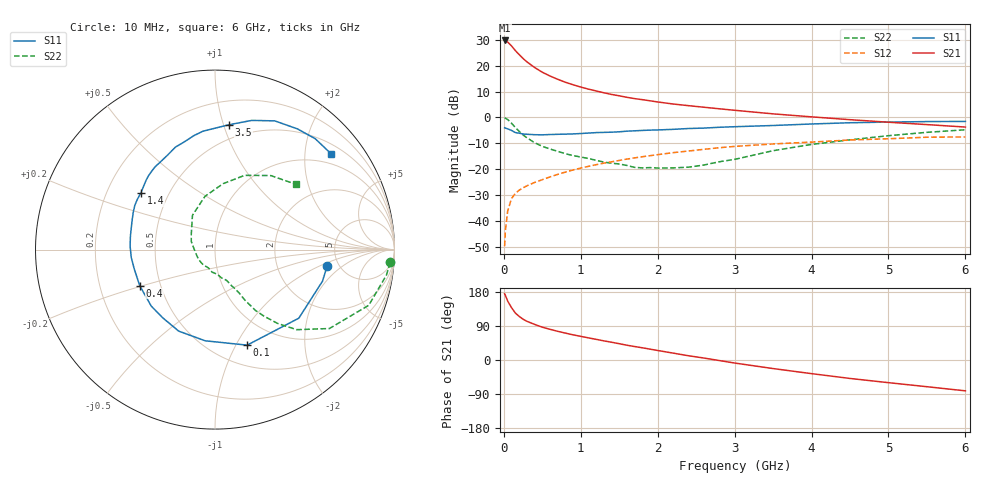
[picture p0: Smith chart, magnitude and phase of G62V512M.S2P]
! SIEMENS Small Signal Semiconductors
! BFG193
! Si NPN RF Bipolar Junction Transistor in SOT223
! VCE = 2.5 V  IC = 12 mA
! Common Emitter S-Parameters:  August  1996
# GHz  S  MA  R  50
!  f  S11  S21  S12  S22
! GHz  MAG  ANG  MAG  ANG  MAG  ANG  MAG  ANG
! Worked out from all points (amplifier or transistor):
!   36 points, 10 MHz to 6 GHz, reference 50 ohm
!   highest |S21| = 29.7 dB at 10 MHz (marker M1)
!   |S21| within 3 dB of that: start of sweep to 124.6 MHz
!   unconditionally stable (mu >= 1): 802.7 MHz to 2.628 GHz
!   at 250 MHz: K = 0.60, MSG = 24.9 dB, |S12| = -27.1 dB
!   at 1.4 GHz: K = 1.07, MAG = 11.4 dB, |S12| = -17.1 dB
!   at 6 GHz: K = 0.90, MSG = 1.9 dB, |S12| = -7.5 dB
!   S11 on the Smith chart (normalised r, x): 10 MHz: 4.05, -1.22; 100 MHz: 0.72, -1.11; 400 MHz: 0.38, -0.20; 1.4 GHz: 0.35, +0.30; 3.5 GHz: 0.38, +1.04; 6 GHz: 0.72, +2.61
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0.01  0.632 -8.2  30.51 174.7  0.0033 88.0  0.9787 -4.2
0.02  0.6242 -16.4  30.2 170.5  0.0066 84.7  0.966 -8.4
0.05  0.6034 -39.3  28.38 155.4  0.0157 73.2  0.9112 -19.9
0.1  0.5616 -71.4  23.92 138.1  0.0274 62.9  0.7744 -34.6
0.15  0.5111 -96.1  19.44 123.8  0.0344 55.8  0.6376 -44.4
0.2  0.4972 -114.0  16.25 115.0  0.0397 53.2  0.5396 -49.7
0.25  0.4787 -127.6  13.7 107.6  0.044 51.5  0.4595 -53.7
0.3  0.4746 -138.5  11.8 102.1  0.0481 51.7  0.4063 -56.4
0.4  0.4651 -154.4  9.191 93.9  0.0558 52.2  0.3259 -59.4
0.5  0.4625 -166.3  7.444 86.6  0.0631 52.0  0.2771 -60.9
0.6  0.4686 -174.6  6.301 81.0  0.0715 52.6  0.2464 -62.7
0.7  0.4733 177.7  5.442 75.7  0.0799 52.8  0.2223 -65.3
0.9  0.4815 165.8  4.267 66.4  0.0973 51.8  0.1839 -69.2
1.1  0.5003 155.6  3.516 58.4  0.1142 50.3  0.1616 -77.1
1.4  0.5199 142.5  2.776 46.9  0.1396 46.1  0.1314 -90.6
1.7  0.5528 132.3  2.308 35.5  0.1661 41.6  0.1091 -108.5
2.2  0.5899 116.4  1.818 18.2  0.2095 31.9  0.1066 -150.5
2.8  0.6463 100.4  1.469 -1.4  0.2607 19.4  0.1398 160.9
3.5  0.6996 83.7  1.173 -22.6  0.3083 2.9  0.2287 123.3
4.5  0.7907 65.1  0.906 -48.7  0.3678 -16.8  0.37 83.0
5.5  0.8327 47.9  0.728 -70.5  0.4158 -40.5  0.5165 53.0
6  0.8388 39.5  0.653 -81.4  0.4214 -54.1  0.5787 39.0
